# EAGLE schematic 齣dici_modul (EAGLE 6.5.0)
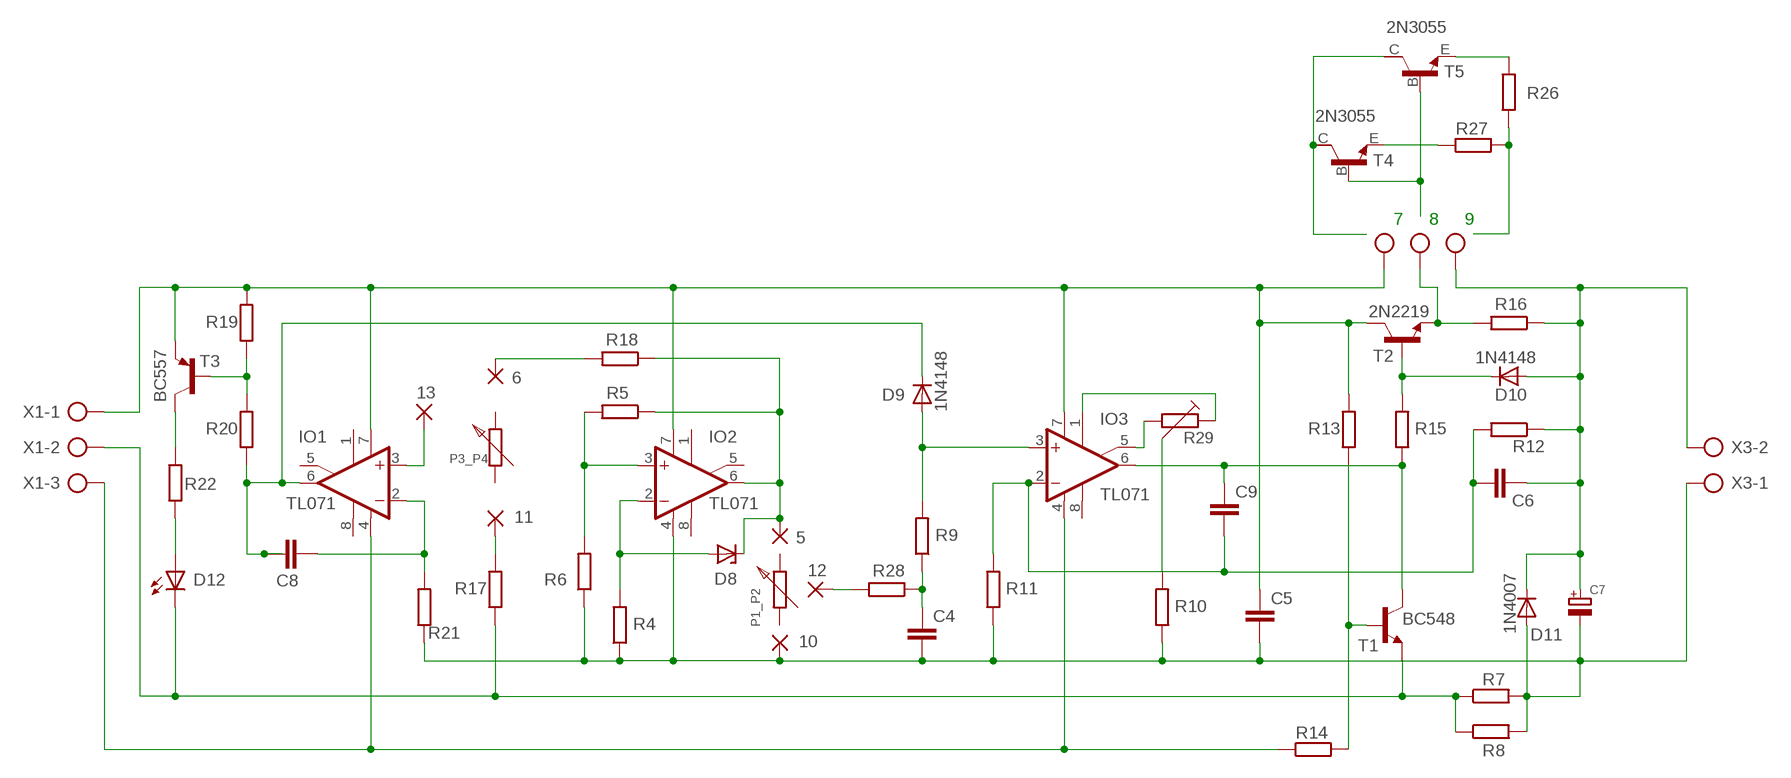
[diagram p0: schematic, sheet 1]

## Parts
5  WIREPAD2,54/1,0  [2,54/1,0]
6  WIREPAD2,54/1,0  [2,54/1,0]
8  8  AK500/3-H  [AK500/3-H]
10  WIREPAD2,54/1,0  [2,54/1,0]
11  WIREPAD2,54/1,0  [2,54/1,0]
12  WIREPAD2,54/1,0  [2,54/1,0]
13  WIREPAD2,54/1,0  [2,54/1,0]
C4  CK  [C3X5]
C5  WIMA-RM5-3,5  [C5-3,5X7]
C6  CK  [C3X5]
C7  ELETKROLYT-5X10-RAD  [ELYT-5RM_10MM/RAD]
C8  CK  [C3X5]
C9  CK  [C3X5]
D8  BZX85  [DO41Z10]
D9  1N4148  [DO35-10]
D10  1N4148  [DO35-10]
D11  1N4007  [DO41-10]
D12  LED5MM  [LED5MM]
IO1  TL071  TL071P  [DIL08]
IO2  TL071  TL071P  [DIL08]
IO3  TL071  TL071P  [DIL08]
P1_P2  POTENCIOMETR  [POT-15MM_RM10_MONO]
P3_P4  POTENCIOMETR  [POT-15MM_RM10_MONO]
R4  R-EU_0207/7  [0207/7]
R5  R-EU_0207/7  [0207/7]
R6  R-EU_0207/7  [0207/7]
R7  R-EU_0922/22  [0922/22]
R8  R-EU_0922/22  [0922/22]
R9  R-EU_0207/7  [0207/7]
R10  R-EU_0207/7  [0207/7]
R11  R-EU_0207/7  [0207/7]
R12  R-EU_0207/7  [0207/7]
R13  R-EU_0207/7  [0207/7]
R14  R-EU_0207/7  [0207/7]
R15  R-EU_0207/7  [0207/7]
R16  R-EU_0207/7  [0207/7]
R17  R-EU_0207/7  [0207/7]
R18  R-EU_0207/7  [0207/7]
R19  R-EU_0207/7  [0207/7]
R20  R-EU_0207/7  [0207/7]
R21  R-EU_0207/7  [0207/7]
R22  R-EU_0207/7  [0207/7]
R26  R-EU_0207/7  [0207/7]
R27  R-EU_0207/7  [0207/7]
R28  R-EU_0207/7  [0207/7]
R29  PT-6_V-LEZ  [PT6V]
T1  BC548  [TO92-EBC]
T2  2N2219  [TO5]
T3  BC557  [TO92]
T4  2N3055  [TO3]
T5  2N3055  [TO3]
X1  AK500/3-H  [AK500/3-H]
X3  AK500/2-H  [AK500/2-H]

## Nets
N$1: 8.3 C5.1 IO1.7(V+) IO2.7(V+) IO3.7(V+) R13.2 R19.2 T2.3(C) T3.1(E) X1.1
N$2: R22.2 T3.3(C)
N$3: D12.A R22.1
N$4: IO3.5(ON2) R29.2
N$5: IO1.4(V-) IO3.4(V-) R14.1 X1.3
N$6: R19.1 R20.2 T3.2(B)
N$7: C8.1 D9.C IO1.6(OUT) R20.1
N$8: C8.2 IO1.2(-IN) R21.2
N$9: 13.1(P) IO1.3(+IN)
N$10: 11.1(P) R17.2
N$11: 12.1(P) R28.2
N$12: D8.A IO2.2(-IN) R4.2
N$13: IO2.3(+IN) R5.2 R6.2
N$14: 6.1(P) R18.2
N$15: 5.1(P) D8.C IO2.6(OUT) R5.1 R18.1
N$16: R10.2 R29.3
N$18: C4.1 R9.1 R28.1
N$19: D9.A IO3.3(+IN) R9.2
N$20: C6.1 C9.2 IO3.2(-IN) R11.2 R12.2
N$21: IO3.1(ON1) R29.1
N$22: C9.1 IO3.6(OUT) R15.1 T1.C
N$23: 8.2 R16.2 T2.1(E)
N$24: R13.1 R14.2 T1.B
N$25: 8.1 C6.2 C7.P$1(+) D10.A D11.C R12.1 R16.1 X3.2
N$26: D10.C R15.2 T2.2(B)
N$27: 10.1(P) C4.2 C5.2 C7.P$2(-) D11.A IO2.4(V-) R4.1 R6.1 R7.2 R8.2 R10.1 R11.1 R21.1 X3.1
N$28: D12.K(C) R7.1 R8.1 R17.1 T1.E X1.2
N$29: R26.1 T5.E
N$30: R26.2 R27.2
N$31: R27.1 T4.E
N$32: T4.B T5.B
N$33: T4.C T5.C
Unconnected: IO1.1(ON1) IO1.5(ON2) IO1.8(OPT) IO2.1(ON1) IO2.5(ON2) IO2.8(OPT) IO3.8(OPT) P1_P2.1 P1_P2.2 P1_P2.3 P3_P4.1 P3_P4.2 P3_P4.3 T4.C/(C) T5.C/(C)

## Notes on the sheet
- 7 | 8 | 9

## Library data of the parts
5 6 10-13 = wirepad:WIREPAD: Wire PAD connect wire on PCB
8 X1 = con-ptr500:AK500/3-H: CONNECTOR Aug. 2004 / PTR Meßtechnik: Die Bezeichnung der Serie AK505 wurde geändert. Es handelt sich hierbei um AK500 in horizontaler Ausführung.; OC_FARNELL: unknown; OC_NEWARK: unknown
C4 C6 C8 C9 = kondenzatory:CK: Keramické kondenzátory rady CK
C5 = kondenzatory:WIMA-RM5: Kondenzátory fóliové WIMA RM 5
C7 = Kondenzátory:ELETKROLYT: ELEKTROLYTICKÝ KONDENZÁTOR
D8 = diode:BZX85: Z DIODE
D9 D10 = diody:1N4148: Univerzální dioda
D11 = diody:1N4007: Usmernovací dioda
D12 = led:LED: LED
IO1-IO3 = linear:TL071: OP AMP
P1_P2 P3_P4 = Potenciometry, trimry:POTENCIOMETR
R4-R22 R26-R28 = resistor:R-EU_: RESISTOR, European symbol
R29 = #PaJa_21:PT-6: Trimr PT6 - 6,3mm
T1 = transistor-npn:BC548*: NPN Transistor
T2 = tranzistory NPN:2N2219: NPN TRANSISTOR
T3 = transistor-pnp:BC557: PNP Transistor
T4 T5 = transistor-neu-to92:2N3055: NPN TRANSISTOR
X3 = con-ptr500:AK500/2-H: CONNECTOR; OC_FARNELL: unknown; OC_NEWARK: unknown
